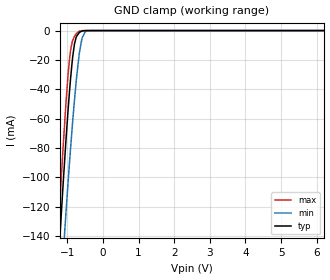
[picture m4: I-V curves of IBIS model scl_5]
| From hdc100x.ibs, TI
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|   scl_5 Model
[Model]   scl_5
Model_type   Input
Vinl = 1.5
Vinh = 3.5
|   typ   min   max
|   (nom PVT)   (fast PVT)   (slow PVT)
C_comp   4.581e-13   4.355e-13   5.484e-13
[Model spec]
|subparameter
Vinl   1.5   1.35   1.65
Vinh   3.5   3.15   3.85
| Where nom  PVT is Nominal Process, 5V, 27C
|   Fast PVT is Strong Process,  5.5V, -40C
|   Slow PVT is Weak Process,   4.5V, 150C
[Voltage Range]   5   4.5   5.5
|Junction Temperature
[Temperature Range]   27   150   -40
[Power Clamp Reference]   5   4.5   5.5
[GND Clamp Reference]   0   0   0
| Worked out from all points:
|   GND clamp passes 1 mA (typ) near -0.64 V on its own axis
[GND Clamp]
|   Voltage   I(typ)   I(min)   I(max)
-5V       -1.919A    -1.85A     -1.968A
-1.288V   -174.9mA   -219.3mA   -152.8mA
-1.224V   -148.4mA   -194.6mA   -124.8mA
-1.12V    -106mA     -154.7mA   -80.8mA
-1.04V    -75.79mA   -125.4mA   -50.41mA
-940mV    -42.29mA   -90.81mA   -20.1mA
-860mV    -20.61mA   -65.41mA   -7.611mA
-800mV    -9.43mA    -47.96mA   -4.074mA
-660.5mV  -1.264mA   -15.15mA   -391.6uA
-585.5mV  -307.9uA   -5.078mA   -51.23uA
-365mV    -932.9nA   -57.1uA    -19.24nA
10V       0A         0A         0A
[POWER Clamp]
|   Voltage   I(typ)   I(min)   I(max)
-5V       0A         0A         0A
0V        0A         0A         0A
10V       0A         0A         0A
